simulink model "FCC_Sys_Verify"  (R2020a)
settings: Solver=FixedStepDiscrete  StartTime=0.0  StopTime=10.0  FixedStep=.001  RelTol=1e-3  EnableMultiTasking=on
undefined symbols (not defined in the file or in its folder): sldvsubsys
libraries: sldvlib x3

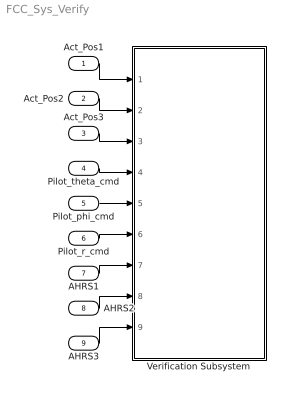
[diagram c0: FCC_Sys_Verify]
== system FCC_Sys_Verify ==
  Act_Pos1 : Inport  OutMin=-32768  OutMax=32767  OutDataTypeStr=int16  PortDimensions=1  SampleTime=0.001
  Act_Pos2 : Inport  Port=2  OutMin=-32768  OutMax=32767  OutDataTypeStr=int16  PortDimensions=1  SampleTime=0.001
  Act_Pos3 : Inport  Port=3  OutMin=-32768  OutMax=32767  OutDataTypeStr=int16  PortDimensions=1  SampleTime=0.001
  Pilot_theta_cmd : Inport  Port=4  OutMin=-32768  OutMax=32767  OutDataTypeStr=int16  PortDimensions=1  SampleTime=0.01
  Pilot_phi_cmd : Inport  Port=5  OutMin=-32768  OutMax=32767  OutDataTypeStr=int16  PortDimensions=1  SampleTime=0.01
  Pilot_r_cmd : Inport  Port=6  OutMin=-32768  OutMax=32767  OutDataTypeStr=int16  PortDimensions=1  SampleTime=0.01
  AHRS1 : Inport  Port=7  OutDataTypeStr=Bus: AHRS_Bus  PortDimensions=1  SampleTime=0.01
  AHRS2 : Inport  Port=8  OutDataTypeStr=Bus: AHRS_Bus  PortDimensions=1  SampleTime=0.01
  AHRS3 : Inport  Port=9  OutDataTypeStr=Bus: AHRS_Bus  PortDimensions=1  SampleTime=0.01
  Verification Subsystem : Subsystem  Tag=VerificationSubsystem  DisableCoverage=on  LoadFcn=sldvsubsys('check')  TreatAsAtomicUnit=on  SimViewingDevice=on  mask(VerificationSubsystem){}
      mask init:
      | sldvsubsys('maskInit');
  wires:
  Act_Pos1/1 -> Verification Subsystem/1(Act_Pos1)
  Act_Pos2/1 -> Verification Subsystem/2(Act_Pos2)
  Act_Pos3/1 -> Verification Subsystem/3(Act_Pos3)
  Pilot_theta_cmd/1 -> Verification Subsystem/4(Pilot_theta_cmd)
  Pilot_phi_cmd/1 -> Verification Subsystem/5(Pilot_phi_cmd)
  Pilot_r_cmd/1 -> Verification Subsystem/6(Pilot_r_cmd)
  AHRS1/1 -> Verification Subsystem/7(AHRS1)
  AHRS2/1 -> Verification Subsystem/8(AHRS2)
  AHRS3/1 -> Verification Subsystem/9(AHRS3)

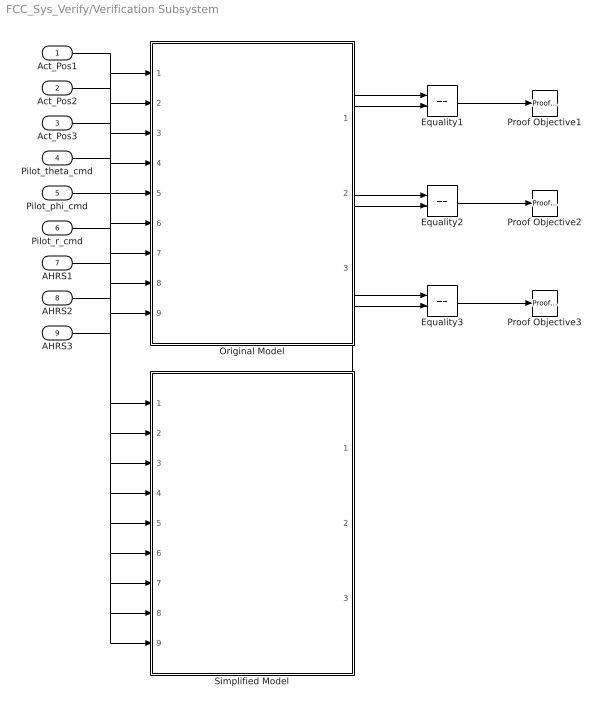
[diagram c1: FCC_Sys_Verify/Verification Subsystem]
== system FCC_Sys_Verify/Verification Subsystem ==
  Act_Pos1 : Inport  OutMin=-32768  OutMax=32767  OutDataTypeStr=int16  PortDimensions=1  SampleTime=0.001
  Act_Pos2 : Inport  Port=2  OutMin=-32768  OutMax=32767  OutDataTypeStr=int16  PortDimensions=1  SampleTime=0.001
  Act_Pos3 : Inport  Port=3  OutMin=-32768  OutMax=32767  OutDataTypeStr=int16  PortDimensions=1  SampleTime=0.001
  Pilot_theta_cmd : Inport  Port=4  OutMin=-32768  OutMax=32767  OutDataTypeStr=int16  PortDimensions=1  SampleTime=0.01
  Pilot_phi_cmd : Inport  Port=5  OutMin=-32768  OutMax=32767  OutDataTypeStr=int16  PortDimensions=1  SampleTime=0.01
  Pilot_r_cmd : Inport  Port=6  OutMin=-32768  OutMax=32767  OutDataTypeStr=int16  PortDimensions=1  SampleTime=0.01
  AHRS1 : Inport  Port=7  OutDataTypeStr=Bus: AHRS_Bus  PortDimensions=1  SampleTime=0.01
  AHRS2 : Inport  Port=8  OutDataTypeStr=Bus: AHRS_Bus  PortDimensions=1  SampleTime=0.01
  AHRS3 : Inport  Port=9  OutDataTypeStr=Bus: AHRS_Bus  PortDimensions=1  SampleTime=0.01
  Equality1 : RelationalOperator  Operator===  OutDataTypeStr=boolean  RndMeth=Simplest
  Equality2 : RelationalOperator  Operator===  OutDataTypeStr=boolean  RndMeth=Simplest
  Equality3 : RelationalOperator  Operator===  OutDataTypeStr=boolean  RndMeth=Simplest
  Original Model : ModelReference  ModelNameDialog=FCC_Sys_Original  SimulationMode=Normal  ModelReferenceVersion=1.73
  Proof Objective1 : sldvlib/Objectives and Constraints/Proof Objective  enabled=on  customAVTBlockType=Proof Objective  intervals=true  dispValues=on  outEnabled=off  enableStopSim=off
  Proof Objective2 : sldvlib/Objectives and Constraints/Proof Objective  enabled=on  customAVTBlockType=Proof Objective  intervals=true  dispValues=on  outEnabled=off  enableStopSim=off
  Proof Objective3 : sldvlib/Objectives and Constraints/Proof Objective  enabled=on  customAVTBlockType=Proof Objective  intervals=true  dispValues=on  outEnabled=off  enableStopSim=off
  Simplified Model : ModelReference  ModelNameDialog=FCC_Sys_New  SimulationMode=Normal  ModelReferenceVersion=1.75
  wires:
  Act_Pos1/1 -> Original Model/1, Simplified Model/1
  Act_Pos2/1 -> Original Model/2, Simplified Model/2
  Act_Pos3/1 -> Original Model/3, Simplified Model/3
  Pilot_theta_cmd/1 -> Original Model/4, Simplified Model/4
  Pilot_phi_cmd/1 -> Original Model/5, Simplified Model/5
  Pilot_r_cmd/1 -> Original Model/6, Simplified Model/6
  AHRS1/1 -> Original Model/7, Simplified Model/7
  AHRS2/1 -> Original Model/8, Simplified Model/8
  AHRS3/1 -> Original Model/9, Simplified Model/9
  Original Model/1 -> Equality1/1
  Simplified Model/1 -> Equality1/2
  Equality1/1 -> Proof Objective1/1
  Original Model/2 -> Equality2/1
  Simplified Model/2 -> Equality2/2
  Equality2/1 -> Proof Objective2/1
  Original Model/3 -> Equality3/1
  Simplified Model/3 -> Equality3/2
  Equality3/1 -> Proof Objective3/1
